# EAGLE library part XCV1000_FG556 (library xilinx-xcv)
xcv1000_fg556_1532 edit this description Auto generated by make-symbol-device-package-bsdl.ulp Rev. 26 Source: xcv1000_fg556_1532.bsd
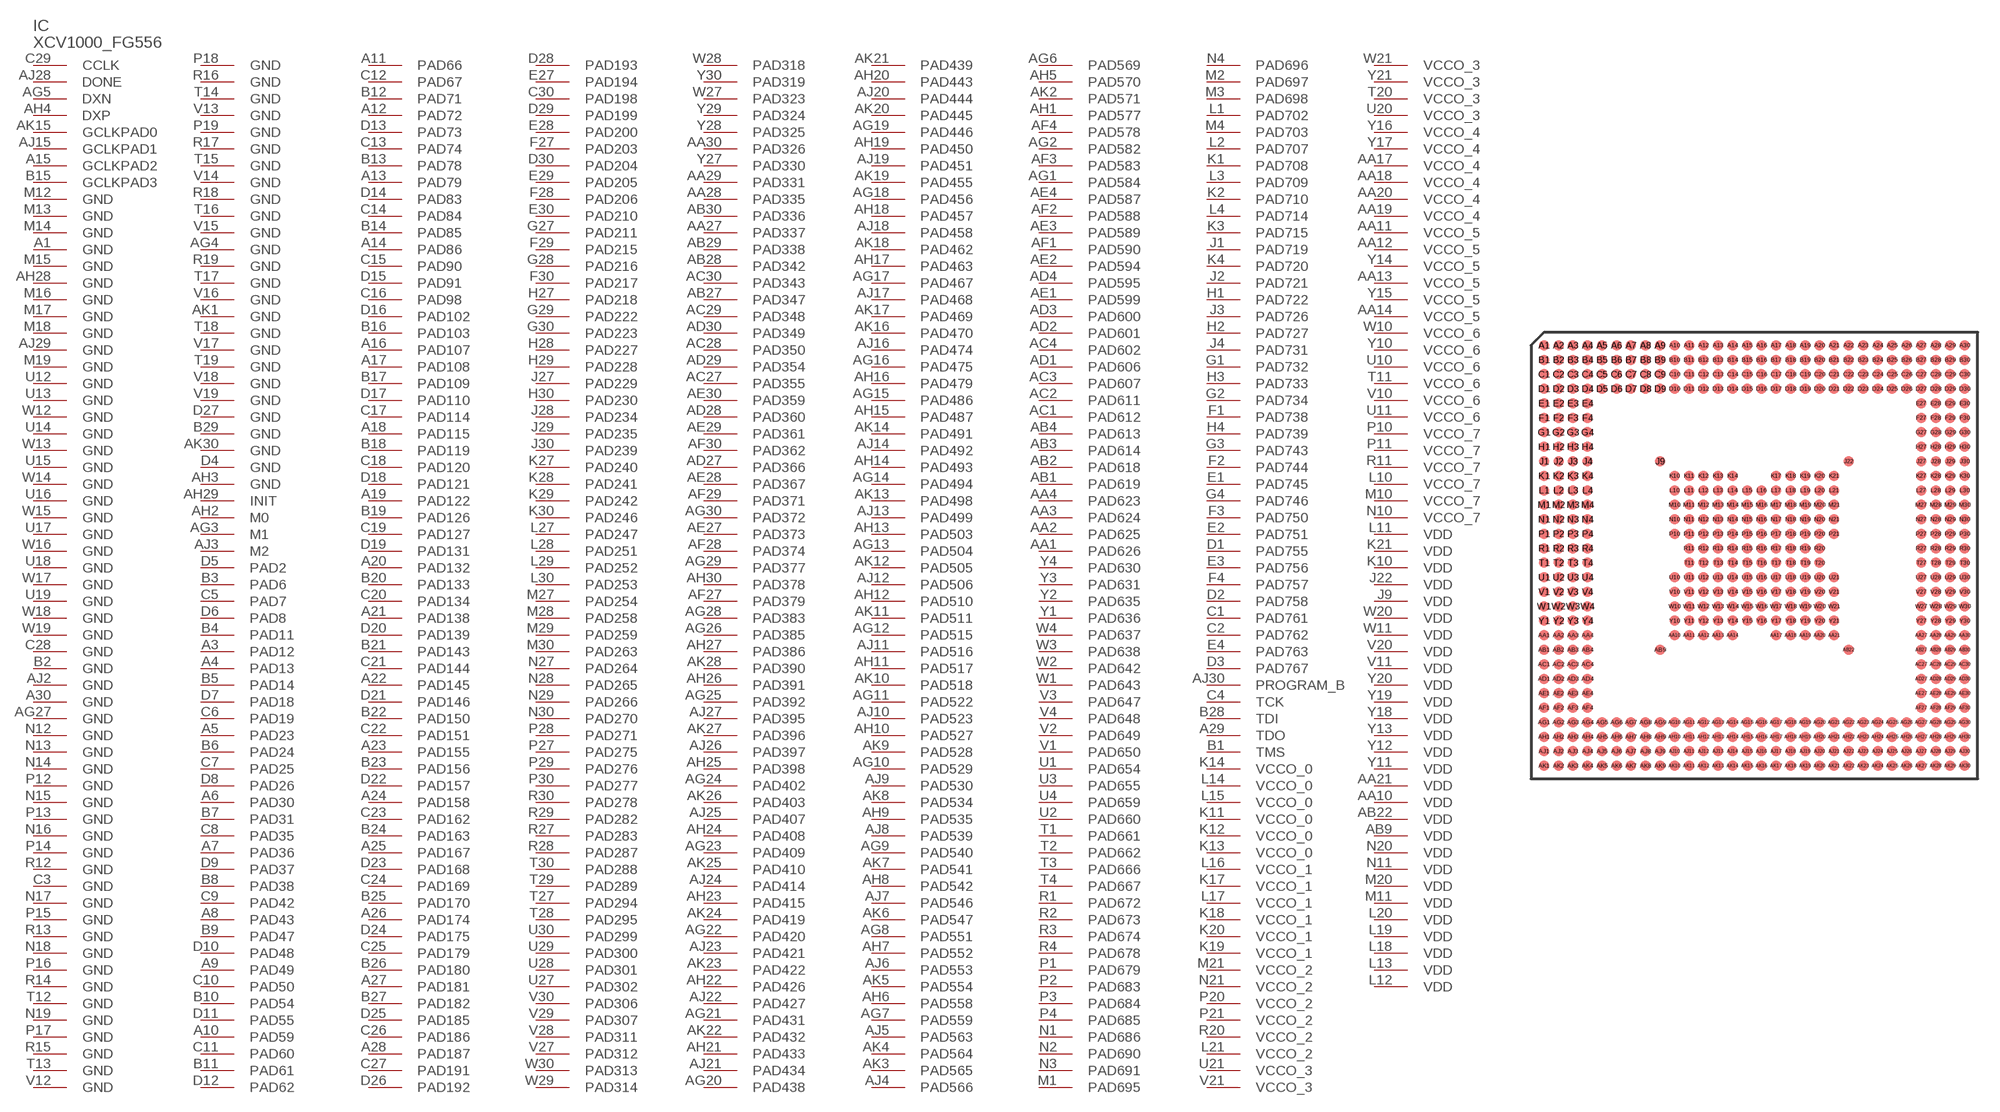
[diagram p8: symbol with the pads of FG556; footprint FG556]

Designator prefix IC

## XCV1000_FG556 (OC_FARNELL: unknown; OC_NEWARK: unknown)  [FG556]
A1  GND  pwr
A3  PAD12
A4  PAD13
A5  PAD23
A6  PAD30
A7  PAD36
A8  PAD43
A9  PAD49
A10  PAD59
A11  PAD66
A12  PAD72
A13  PAD79
A14  PAD86
A15  GCLKPAD2  in
A16  PAD107
A17  PAD108
A18  PAD115
A19  PAD122
A20  PAD132
A21  PAD138
A22  PAD145
A23  PAD155
A24  PAD158
A25  PAD167
A26  PAD174
A27  PAD181
A28  PAD187
A29  TDO  out
A30  GND  pwr
AA1  PAD626
AA2  PAD625
AA3  PAD624
AA4  PAD623
AA10  VDD  pwr
AA11  VCCO_5  pwr
AA12  VCCO_5  pwr
AA13  VCCO_5  pwr
AA14  VCCO_5  pwr
AA17  VCCO_4  pwr
AA18  VCCO_4  pwr
AA19  VCCO_4  pwr
AA20  VCCO_4  pwr
AA21  VDD  pwr
AA27  PAD337
AA28  PAD335
AA29  PAD331
AA30  PAD326
AB1  PAD619
AB2  PAD618
AB3  PAD614
AB4  PAD613
AB9  VDD  pwr
AB22  VDD  pwr
AB27  PAD347
AB28  PAD342
AB29  PAD338
AB30  PAD336
AC1  PAD612
AC2  PAD611
AC3  PAD607
AC4  PAD602
AC27  PAD355
AC28  PAD350
AC29  PAD348
AC30  PAD343
AD1  PAD606
AD2  PAD601
AD3  PAD600
AD4  PAD595
AD27  PAD366
AD28  PAD360
AD29  PAD354
AD30  PAD349
AE1  PAD599
AE2  PAD594
AE3  PAD589
AE4  PAD587
AE27  PAD373
AE28  PAD367
AE29  PAD361
AE30  PAD359
AF1  PAD590
AF2  PAD588
AF3  PAD583
AF4  PAD578
AF27  PAD379
AF28  PAD374
AF29  PAD371
AF30  PAD362
AG1  PAD584
AG2  PAD582
AG3  M1  in
AG4  GND  pwr
AG5  DXN  pas
AG6  PAD569
AG7  PAD559
AG8  PAD551
AG9  PAD540
AG10  PAD529
AG11  PAD522
AG12  PAD515
AG13  PAD504
AG14  PAD494
AG15  PAD486
AG16  PAD475
AG17  PAD467
AG18  PAD456
AG19  PAD446
AG20  PAD438
AG21  PAD431
AG22  PAD420
AG23  PAD409
AG24  PAD402
AG25  PAD392
AG26  PAD385
AG27  GND  pwr
AG28  PAD383
AG29  PAD377
AG30  PAD372
AH1  PAD577
AH2  M0  in
AH3  GND  pwr
AH4  DXP  pas
AH5  PAD570
AH6  PAD558
AH7  PAD552
AH8  PAD542
AH9  PAD535
AH10  PAD527
AH11  PAD517
AH12  PAD510
AH13  PAD503
AH14  PAD493
AH15  PAD487
AH16  PAD479
AH17  PAD463
AH18  PAD457
AH19  PAD450
AH20  PAD443
AH21  PAD433
AH22  PAD426
AH23  PAD415
AH24  PAD408
AH25  PAD398
AH26  PAD391
AH27  PAD386
AH28  GND  pwr
AH29  INIT
AH30  PAD378
AJ2  GND  pwr
AJ3  M2  in
AJ4  PAD566
AJ5  PAD563
AJ6  PAD553
AJ7  PAD546
AJ8  PAD539
AJ9  PAD530
AJ10  PAD523
AJ11  PAD516
AJ12  PAD506
AJ13  PAD499
AJ14  PAD492
AJ15  GCLKPAD1  in
AJ16  PAD474
AJ17  PAD468
AJ18  PAD458
AJ19  PAD451
AJ20  PAD444
AJ21  PAD434
AJ22  PAD427
AJ23  PAD421
AJ24  PAD414
AJ25  PAD407
AJ26  PAD397
AJ27  PAD395
AJ28  DONE
AJ29  GND  pwr
AJ30  PROGRAM_B  in
AK1  GND  pwr
AK2  PAD571
AK3  PAD565
AK4  PAD564
AK5  PAD554
AK6  PAD547
AK7  PAD541
AK8  PAD534
AK9  PAD528
AK10  PAD518
AK11  PAD511
AK12  PAD505
AK13  PAD498
AK14  PAD491
AK15  GCLKPAD0  in
AK16  PAD470
AK17  PAD469
AK18  PAD462
AK19  PAD455
AK20  PAD445
AK21  PAD439
AK22  PAD432
AK23  PAD422
AK24  PAD419
AK25  PAD410
AK26  PAD403
AK27  PAD396
AK28  PAD390
AK30  GND  pwr
B1  TMS  in
B2  GND  pwr
B3  PAD6
B4  PAD11
B5  PAD14
B6  PAD24
B7  PAD31
B8  PAD38
B9  PAD47
B10  PAD54
B11  PAD61
B12  PAD71
B13  PAD78
B14  PAD85
B15  GCLKPAD3  in
B16  PAD103
B17  PAD109
B18  PAD119
B19  PAD126
B20  PAD133
B21  PAD143
B22  PAD150
B23  PAD156
B24  PAD163
B25  PAD170
B26  PAD180
B27  PAD182
B28  TDI  in
B29  GND  pwr
C1  PAD761
C2  PAD762
C3  GND  pwr
C4  TCK  in
C5  PAD7
C6  PAD19
C7  PAD25
C8  PAD35
C9  PAD42
C10  PAD50
C11  PAD60
C12  PAD67
C13  PAD74
C14  PAD84
C15  PAD90
C16  PAD98
C17  PAD114
C18  PAD120
C19  PAD127
C20  PAD134
C21  PAD144
C22  PAD151
C23  PAD162
C24  PAD169
C25  PAD179
C26  PAD186
C27  PAD191
C28  GND  pwr
C29  CCLK
C30  PAD198
D1  PAD755
D2  PAD758
D3  PAD767
D4  GND  pwr
D5  PAD2
D6  PAD8
D7  PAD18
D8  PAD26
D9  PAD37
D10  PAD48
D11  PAD55
D12  PAD62
D13  PAD73
D14  PAD83
D15  PAD91
D16  PAD102
D17  PAD110
D18  PAD121
D19  PAD131
D20  PAD139
D21  PAD146
D22  PAD157
D23  PAD168
D24  PAD175
D25  PAD185
D26  PAD192
D27  GND  pwr
D28  PAD193
D29  PAD199
D30  PAD204
E1  PAD745
E2  PAD751
E3  PAD756
E4  PAD763
E27  PAD194
E28  PAD200
E29  PAD205
E30  PAD210
F1  PAD738
F2  PAD744
F3  PAD750
F4  PAD757
F27  PAD203
F28  PAD206
F29  PAD215
F30  PAD217
G1  PAD732
G2  PAD734
G3  PAD743
G4  PAD746
G27  PAD211
G28  PAD216
G29  PAD222
G30  PAD223
H1  PAD722
H2  PAD727
H3  PAD733
H4  PAD739
H27  PAD218
H28  PAD227
H29  PAD228
H30  PAD230
J1  PAD719
J2  PAD721
J3  PAD726
J4  PAD731
J9  VDD  pwr
J22  VDD  pwr
J27  PAD229
J28  PAD234
J29  PAD235
J30  PAD239
K1  PAD708
K2  PAD710
K3  PAD715
K4  PAD720
K10  VDD  pwr
K11  VCCO_0  pwr
K12  VCCO_0  pwr
K13  VCCO_0  pwr
K14  VCCO_0  pwr
K17  VCCO_1  pwr
K18  VCCO_1  pwr
K19  VCCO_1  pwr
K20  VCCO_1  pwr
K21  VDD  pwr
K27  PAD240
K28  PAD241
K29  PAD242
K30  PAD246
L1  PAD702
L2  PAD707
L3  PAD709
L4  PAD714
L10  VCCO_7  pwr
L11  VDD  pwr
L12  VDD  pwr
L13  VDD  pwr
L14  VCCO_0  pwr
L15  VCCO_0  pwr
L16  VCCO_1  pwr
L17  VCCO_1  pwr
L18  VDD  pwr
L19  VDD  pwr
L20  VDD  pwr
L21  VCCO_2  pwr
L27  PAD247
L28  PAD251
L29  PAD252
L30  PAD253
M1  PAD695
M2  PAD697
M3  PAD698
M4  PAD703
M10  VCCO_7  pwr
M11  VDD  pwr
M12  GND  pwr
M13  GND  pwr
M14  GND  pwr
M15  GND  pwr
M16  GND  pwr
M17  GND  pwr
M18  GND  pwr
M19  GND  pwr
M20  VDD  pwr
M21  VCCO_2  pwr
M27  PAD254
M28  PAD258
M29  PAD259
M30  PAD263
N1  PAD686
N2  PAD690
N3  PAD691
N4  PAD696
N10  VCCO_7  pwr
N11  VDD  pwr
N12  GND  pwr
N13  GND  pwr
N14  GND  pwr
N15  GND  pwr
N16  GND  pwr
N17  GND  pwr
N18  GND  pwr
N19  GND  pwr
N20  VDD  pwr
N21  VCCO_2  pwr
N27  PAD264
N28  PAD265
N29  PAD266
N30  PAD270
P1  PAD679
P2  PAD683
P3  PAD684
P4  PAD685
P10  VCCO_7  pwr
P11  VCCO_7  pwr
P12  GND  pwr
P13  GND  pwr
P14  GND  pwr
P15  GND  pwr
P16  GND  pwr
P17  GND  pwr
P18  GND  pwr
P19  GND  pwr
P20  VCCO_2  pwr
P21  VCCO_2  pwr
P27  PAD275
P28  PAD271
P29  PAD276
P30  PAD277
R1  PAD672
R2  PAD673
R3  PAD674
R4  PAD678
R11  VCCO_7  pwr
R12  GND  pwr
R13  GND  pwr
R14  GND  pwr
R15  GND  pwr
R16  GND  pwr
R17  GND  pwr
R18  GND  pwr
R19  GND  pwr
R20  VCCO_2  pwr
R27  PAD283
R28  PAD287
R29  PAD282
R30  PAD278
T1  PAD661
T2  PAD662
T3  PAD666
T4  PAD667
T11  VCCO_6  pwr
T12  GND  pwr
T13  GND  pwr
T14  GND  pwr
T15  GND  pwr
T16  GND  pwr
T17  GND  pwr
T18  GND  pwr
T19  GND  pwr
T20  VCCO_3  pwr
T27  PAD294
T28  PAD295
T29  PAD289
T30  PAD288
U1  PAD654
U2  PAD660
U3  PAD655
U4  PAD659
U10  VCCO_6  pwr
U11  VCCO_6  pwr
U12  GND  pwr
U13  GND  pwr
U14  GND  pwr
U15  GND  pwr
U16  GND  pwr
U17  GND  pwr
U18  GND  pwr
U19  GND  pwr
U20  VCCO_3  pwr
U21  VCCO_3  pwr
U27  PAD302
U28  PAD301
U29  PAD300
U30  PAD299
V1  PAD650
V2  PAD649
V3  PAD647
V4  PAD648
V10  VCCO_6  pwr
V11  VDD  pwr
V12  GND  pwr
V13  GND  pwr
V14  GND  pwr
V15  GND  pwr
V16  GND  pwr
V17  GND  pwr
V18  GND  pwr
V19  GND  pwr
V20  VDD  pwr
V21  VCCO_3  pwr
V27  PAD312
V28  PAD311
V29  PAD307
V30  PAD306
W1  PAD643
W2  PAD642
W3  PAD638
W4  PAD637
W10  VCCO_6  pwr
W11  VDD  pwr
W12  GND  pwr
W13  GND  pwr
W14  GND  pwr
W15  GND  pwr
W16  GND  pwr
W17  GND  pwr
W18  GND  pwr
W19  GND  pwr
W20  VDD  pwr
W21  VCCO_3  pwr
W27  PAD323
W28  PAD318
W29  PAD314
W30  PAD313
Y1  PAD636
Y2  PAD635
Y3  PAD631
Y4  PAD630
Y10  VCCO_6  pwr
Y11  VDD  pwr
Y12  VDD  pwr
Y13  VDD  pwr
Y14  VCCO_5  pwr
Y15  VCCO_5  pwr
Y16  VCCO_4  pwr
Y17  VCCO_4  pwr
Y18  VDD  pwr
Y19  VDD  pwr
Y20  VDD  pwr
Y21  VCCO_3  pwr
Y27  PAD330
Y28  PAD325
Y29  PAD324
Y30  PAD319

## Footprint FG556 (pad centres in mm)
xcv1000_fg556_1532 edit this description Auto generated by make-symbol-device-package-bsdl.ulp Rev. 26 Source: xcv1000_fg556_1532.bsd
smd 0.7 x 0.7: A1 -14.5,14.5; A2 -13.5,14.5; A3 -12.5,14.5; A4 -11.5,14.5; A5 -10.5,14.5; A6 -9.5,14.5; A7 -8.5,14.5; A8 -7.5,14.5; A9 -6.5,14.5; A10 -5.5,14.5; A11 -4.5,14.5; A12 -3.5,14.5; A13 -2.5,14.5; A14 -1.5,14.5; A15 -0.5,14.5; A16 0.5,14.5; A17 1.5,14.5; A18 2.5,14.5; A19 3.5,14.5; A20 4.5,14.5; A21 5.5,14.5; A22 6.5,14.5; A23 7.5,14.5; A24 8.5,14.5; A25 9.5,14.5; A26 10.5,14.5; A27 11.5,14.5; A28 12.5,14.5; A29 13.5,14.5; A30 14.5,14.5; AA1 -14.5,-5.5; AA2 -13.5,-5.5; AA3 -12.5,-5.5; AA4 -11.5,-5.5; AA10 -5.5,-5.5; AA11 -4.5,-5.5; AA12 -3.5,-5.5; AA13 -2.5,-5.5; AA14 -1.5,-5.5; AA17 1.5,-5.5; AA18 2.5,-5.5; AA19 3.5,-5.5; AA20 4.5,-5.5; AA21 5.5,-5.5; AA27 11.5,-5.5; AA28 12.5,-5.5; AA29 13.5,-5.5; AA30 14.5,-5.5; AB1 -14.5,-6.5; AB2 -13.5,-6.5; AB3 -12.5,-6.5; AB4 -11.5,-6.5; AB9 -6.5,-6.5; AB22 6.5,-6.5; AB27 11.5,-6.5; AB28 12.5,-6.5; AB29 13.5,-6.5; AB30 14.5,-6.5; AC1 -14.5,-7.5; AC2 -13.5,-7.5; AC3 -12.5,-7.5; AC4 -11.5,-7.5; AC27 11.5,-7.5; AC28 12.5,-7.5; AC29 13.5,-7.5; AC30 14.5,-7.5; AD1 -14.5,-8.5; AD2 -13.5,-8.5; AD3 -12.5,-8.5; AD4 -11.5,-8.5; AD27 11.5,-8.5; AD28 12.5,-8.5; AD29 13.5,-8.5; AD30 14.5,-8.5; AE1 -14.5,-9.5; AE2 -13.5,-9.5; AE3 -12.5,-9.5; AE4 -11.5,-9.5; AE27 11.5,-9.5; AE28 12.5,-9.5; AE29 13.5,-9.5; AE30 14.5,-9.5; AF1 -14.5,-10.5; AF2 -13.5,-10.5; AF3 -12.5,-10.5; AF4 -11.5,-10.5; AF27 11.5,-10.5; AF28 12.5,-10.5; AF29 13.5,-10.5; AF30 14.5,-10.5; AG1 -14.5,-11.5; AG2 -13.5,-11.5; AG3 -12.5,-11.5; AG4 -11.5,-11.5; AG5 -10.5,-11.5; AG6 -9.5,-11.5; AG7 -8.5,-11.5; AG8 -7.5,-11.5; AG9 -6.5,-11.5; AG10 -5.5,-11.5; AG11 -4.5,-11.5; AG12 -3.5,-11.5; AG13 -2.5,-11.5; AG14 -1.5,-11.5; AG15 -0.5,-11.5; AG16 0.5,-11.5; AG17 1.5,-11.5; AG18 2.5,-11.5; AG19 3.5,-11.5; AG20 4.5,-11.5; AG21 5.5,-11.5; AG22 6.5,-11.5; AG23 7.5,-11.5; AG24 8.5,-11.5; AG25 9.5,-11.5; AG26 10.5,-11.5; AG27 11.5,-11.5; AG28 12.5,-11.5; AG29 13.5,-11.5; AG30 14.5,-11.5; AH1 -14.5,-12.5; AH2 -13.5,-12.5; AH3 -12.5,-12.5; AH4 -11.5,-12.5; AH5 -10.5,-12.5; AH6 -9.5,-12.5; AH7 -8.5,-12.5; AH8 -7.5,-12.5; AH9 -6.5,-12.5; AH10 -5.5,-12.5; AH11 -4.5,-12.5; AH12 -3.5,-12.5; AH13 -2.5,-12.5; AH14 -1.5,-12.5; AH15 -0.5,-12.5; AH16 0.5,-12.5; AH17 1.5,-12.5; AH18 2.5,-12.5; AH19 3.5,-12.5; AH20 4.5,-12.5; AH21 5.5,-12.5; AH22 6.5,-12.5; AH23 7.5,-12.5; AH24 8.5,-12.5; AH25 9.5,-12.5; AH26 10.5,-12.5; AH27 11.5,-12.5; AH28 12.5,-12.5; AH29 13.5,-12.5; AH30 14.5,-12.5; AJ1 -14.5,-13.5; AJ2 -13.5,-13.5; AJ3 -12.5,-13.5; AJ4 -11.5,-13.5; AJ5 -10.5,-13.5; AJ6 -9.5,-13.5; AJ7 -8.5,-13.5; AJ8 -7.5,-13.5; AJ9 -6.5,-13.5; AJ10 -5.5,-13.5; AJ11 -4.5,-13.5; AJ12 -3.5,-13.5; AJ13 -2.5,-13.5; AJ14 -1.5,-13.5; AJ15 -0.5,-13.5; AJ16 0.5,-13.5; AJ17 1.5,-13.5; AJ18 2.5,-13.5; AJ19 3.5,-13.5; AJ20 4.5,-13.5; AJ21 5.5,-13.5; AJ22 6.5,-13.5; AJ23 7.5,-13.5; AJ24 8.5,-13.5; AJ25 9.5,-13.5; AJ26 10.5,-13.5; AJ27 11.5,-13.5; AJ28 12.5,-13.5; AJ29 13.5,-13.5; AJ30 14.5,-13.5; AK1 -14.5,-14.5; AK2 -13.5,-14.5; AK3 -12.5,-14.5; AK4 -11.5,-14.5; AK5 -10.5,-14.5; AK6 -9.5,-14.5; AK7 -8.5,-14.5; AK8 -7.5,-14.5; AK9 -6.5,-14.5; AK10 -5.5,-14.5; AK11 -4.5,-14.5; AK12 -3.5,-14.5; AK13 -2.5,-14.5; AK14 -1.5,-14.5; AK15 -0.5,-14.5; AK16 0.5,-14.5; AK17 1.5,-14.5; AK18 2.5,-14.5; AK19 3.5,-14.5; AK20 4.5,-14.5; AK21 5.5,-14.5; AK22 6.5,-14.5; AK23 7.5,-14.5; AK24 8.5,-14.5; AK25 9.5,-14.5; AK26 10.5,-14.5; AK27 11.5,-14.5; AK28 12.5,-14.5; AK29 13.5,-14.5; AK30 14.5,-14.5; B1 -14.5,13.5; B2 -13.5,13.5; B3 -12.5,13.5; B4 -11.5,13.5; B5 -10.5,13.5; B6 -9.5,13.5; B7 -8.5,13.5; B8 -7.5,13.5; B9 -6.5,13.5; B10 -5.5,13.5; B11 -4.5,13.5; B12 -3.5,13.5; B13 -2.5,13.5; B14 -1.5,13.5; B15 -0.5,13.5; B16 0.5,13.5; B17 1.5,13.5; B18 2.5,13.5; B19 3.5,13.5; B20 4.5,13.5; B21 5.5,13.5; B22 6.5,13.5; B23 7.5,13.5; B24 8.5,13.5; B25 9.5,13.5; B26 10.5,13.5; B27 11.5,13.5; B28 12.5,13.5; B29 13.5,13.5; B30 14.5,13.5; C1 -14.5,12.5; C2 -13.5,12.5; C3 -12.5,12.5; C4 -11.5,12.5; C5 -10.5,12.5; C6 -9.5,12.5; C7 -8.5,12.5; C8 -7.5,12.5; C9 -6.5,12.5; C10 -5.5,12.5; C11 -4.5,12.5; C12 -3.5,12.5; C13 -2.5,12.5; C14 -1.5,12.5; C15 -0.5,12.5; C16 0.5,12.5; C17 1.5,12.5; C18 2.5,12.5; C19 3.5,12.5; C20 4.5,12.5; C21 5.5,12.5; C22 6.5,12.5; C23 7.5,12.5; C24 8.5,12.5; C25 9.5,12.5; C26 10.5,12.5; C27 11.5,12.5; C28 12.5,12.5; C29 13.5,12.5; C30 14.5,12.5; D1 -14.5,11.5; D2 -13.5,11.5; D3 -12.5,11.5; D4 -11.5,11.5; D5 -10.5,11.5; D6 -9.5,11.5; D7 -8.5,11.5; D8 -7.5,11.5; D9 -6.5,11.5; D10 -5.5,11.5; D11 -4.5,11.5; D12 -3.5,11.5; D13 -2.5,11.5; D14 -1.5,11.5; D15 -0.5,11.5; D16 0.5,11.5; D17 1.5,11.5; D18 2.5,11.5; D19 3.5,11.5; D20 4.5,11.5; D21 5.5,11.5; D22 6.5,11.5; D23 7.5,11.5; D24 8.5,11.5; D25 9.5,11.5; D26 10.5,11.5; D27 11.5,11.5; D28 12.5,11.5; D29 13.5,11.5; D30 14.5,11.5; E1 -14.5,10.5; E2 -13.5,10.5; E3 -12.5,10.5; E4 -11.5,10.5; E27 11.5,10.5; E28 12.5,10.5; E29 13.5,10.5; E30 14.5,10.5; F1 -14.5,9.5; F2 -13.5,9.5; F3 -12.5,9.5; F4 -11.5,9.5; F27 11.5,9.5; F28 12.5,9.5; F29 13.5,9.5; F30 14.5,9.5; G1 -14.5,8.5; G2 -13.5,8.5; G3 -12.5,8.5; G4 -11.5,8.5; G27 11.5,8.5; G28 12.5,8.5; G29 13.5,8.5; G30 14.5,8.5; H1 -14.5,7.5; H2 -13.5,7.5; H3 -12.5,7.5; H4 -11.5,7.5; H27 11.5,7.5; H28 12.5,7.5; H29 13.5,7.5; H30 14.5,7.5; J1 -14.5,6.5; J2 -13.5,6.5; J3 -12.5,6.5; J4 -11.5,6.5; J9 -6.5,6.5; J22 6.5,6.5; J27 11.5,6.5; J28 12.5,6.5; J29 13.5,6.5; J30 14.5,6.5; K1 -14.5,5.5; K2 -13.5,5.5; K3 -12.5,5.5; K4 -11.5,5.5; K10 -5.5,5.5; K11 -4.5,5.5; K12 -3.5,5.5; K13 -2.5,5.5; K14 -1.5,5.5; K17 1.5,5.5; K18 2.5,5.5; K19 3.5,5.5; K20 4.5,5.5; K21 5.5,5.5; K27 11.5,5.5; K28 12.5,5.5; K29 13.5,5.5; K30 14.5,5.5; L1 -14.5,4.5; L2 -13.5,4.5; L3 -12.5,4.5; L4 -11.5,4.5; L10 -5.5,4.5; L11 -4.5,4.5; L12 -3.5,4.5; L13 -2.5,4.5; L14 -1.5,4.5; L15 -0.5,4.5; L16 0.5,4.5; L17 1.5,4.5; L18 2.5,4.5; L19 3.5,4.5; L20 4.5,4.5; L21 5.5,4.5; L27 11.5,4.5; L28 12.5,4.5; L29 13.5,4.5; L30 14.5,4.5; M1 -14.5,3.5; M2 -13.5,3.5; M3 -12.5,3.5; M4 -11.5,3.5; M10 -5.5,3.5; M11 -4.5,3.5; M12 -3.5,3.5; M13 -2.5,3.5; M14 -1.5,3.5; M15 -0.5,3.5; M16 0.5,3.5; M17 1.5,3.5; M18 2.5,3.5; M19 3.5,3.5; M20 4.5,3.5; M21 5.5,3.5; M27 11.5,3.5; M28 12.5,3.5; M29 13.5,3.5; M30 14.5,3.5; N1 -14.5,2.5; N2 -13.5,2.5; N3 -12.5,2.5; N4 -11.5,2.5; N10 -5.5,2.5; N11 -4.5,2.5; N12 -3.5,2.5; N13 -2.5,2.5; N14 -1.5,2.5; N15 -0.5,2.5; N16 0.5,2.5; N17 1.5,2.5; N18 2.5,2.5; N19 3.5,2.5; N20 4.5,2.5; N21 5.5,2.5; N27 11.5,2.5; N28 12.5,2.5; N29 13.5,2.5; N30 14.5,2.5; P1 -14.5,1.5; P2 -13.5,1.5; P3 -12.5,1.5; P4 -11.5,1.5; P10 -5.5,1.5; P11 -4.5,1.5; P12 -3.5,1.5; P13 -2.5,1.5; P14 -1.5,1.5; P15 -0.5,1.5; P16 0.5,1.5; P17 1.5,1.5; P18 2.5,1.5; P19 3.5,1.5; P20 4.5,1.5; P21 5.5,1.5; P27 11.5,1.5; P28 12.5,1.5; P29 13.5,1.5; P30 14.5,1.5; R1 -14.5,0.5; R2 -13.5,0.5; R3 -12.5,0.5; R4 -11.5,0.5; R11 -4.5,0.5; R12 -3.5,0.5; R13 -2.5,0.5; R14 -1.5,0.5; R15 -0.5,0.5; R16 0.5,0.5; R17 1.5,0.5; R18 2.5,0.5; R19 3.5,0.5; R20 4.5,0.5; R27 11.5,0.5; R28 12.5,0.5; R29 13.5,0.5; R30 14.5,0.5; T1 -14.5,-0.5; T2 -13.5,-0.5; T3 -12.5,-0.5; T4 -11.5,-0.5; T11 -4.5,-0.5; T12 -3.5,-0.5; T13 -2.5,-0.5; T14 -1.5,-0.5; T15 -0.5,-0.5; T16 0.5,-0.5; T17 1.5,-0.5; T18 2.5,-0.5; T19 3.5,-0.5; T20 4.5,-0.5; T27 11.5,-0.5; T28 12.5,-0.5; T29 13.5,-0.5; T30 14.5,-0.5; U1 -14.5,-1.5; U2 -13.5,-1.5; U3 -12.5,-1.5; U4 -11.5,-1.5; U10 -5.5,-1.5; U11 -4.5,-1.5; U12 -3.5,-1.5; U13 -2.5,-1.5; U14 -1.5,-1.5; U15 -0.5,-1.5; U16 0.5,-1.5; U17 1.5,-1.5; U18 2.5,-1.5; U19 3.5,-1.5; U20 4.5,-1.5; U21 5.5,-1.5; U27 11.5,-1.5; U28 12.5,-1.5; U29 13.5,-1.5; U30 14.5,-1.5; V1 -14.5,-2.5; V2 -13.5,-2.5; V3 -12.5,-2.5; V4 -11.5,-2.5; V10 -5.5,-2.5; V11 -4.5,-2.5; V12 -3.5,-2.5; V13 -2.5,-2.5; V14 -1.5,-2.5; V15 -0.5,-2.5; V16 0.5,-2.5; V17 1.5,-2.5; V18 2.5,-2.5; V19 3.5,-2.5; V20 4.5,-2.5; V21 5.5,-2.5; V27 11.5,-2.5; V28 12.5,-2.5; V29 13.5,-2.5; V30 14.5,-2.5; W1 -14.5,-3.5; W2 -13.5,-3.5; W3 -12.5,-3.5; W4 -11.5,-3.5; W10 -5.5,-3.5; W11 -4.5,-3.5; W12 -3.5,-3.5; W13 -2.5,-3.5; W14 -1.5,-3.5; W15 -0.5,-3.5; W16 0.5,-3.5; W17 1.5,-3.5; W18 2.5,-3.5; W19 3.5,-3.5; W20 4.5,-3.5; W21 5.5,-3.5; W27 11.5,-3.5; W28 12.5,-3.5; W29 13.5,-3.5; W30 14.5,-3.5; Y1 -14.5,-4.5; Y2 -13.5,-4.5; Y3 -12.5,-4.5; Y4 -11.5,-4.5; Y10 -5.5,-4.5; Y11 -4.5,-4.5; Y12 -3.5,-4.5; Y13 -2.5,-4.5; Y14 -1.5,-4.5; Y15 -0.5,-4.5; Y16 0.5,-4.5; Y17 1.5,-4.5; Y18 2.5,-4.5; Y19 3.5,-4.5; Y20 4.5,-4.5; Y21 5.5,-4.5; Y27 11.5,-4.5; Y28 12.5,-4.5; Y29 13.5,-4.5; Y30 14.5,-4.5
